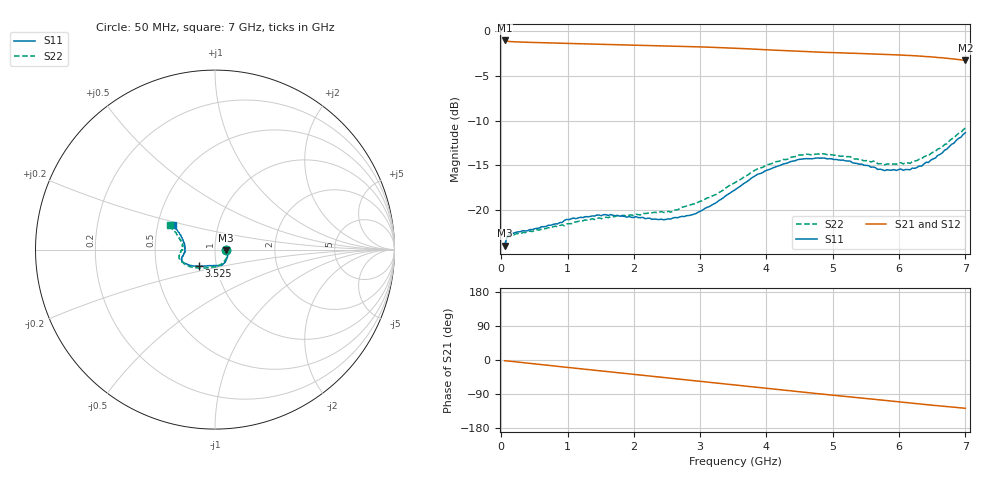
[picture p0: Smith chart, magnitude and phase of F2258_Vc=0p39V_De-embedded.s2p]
! Integrated Device Technology
! Corporate Headquarters
! 6024 Silver Creek Valley Road
! San Jose, CA 95138  USA
! Phone:  1-408-284-8200
! Toll Free:  1-800-223-1366
! Webpage:  http://www.idt.com/
! Timing and RF Division
! 515 Groton Road, Suite 102
! Westford, MA 01886-6024
! Device:  F2258
! Description: Voltage Variable RF Attenuator
! Frequency:  50.0 -  6000.00 MHz
! Package:  3x3 mm Thin QFN Plastic Package: 16 pin
! Ports:  2 RF, 2 DC
!  Pin  1  = NC
!  Pin  2  = NC
!  Pin  3  = RF2  = Port 2
!  Pin  4  = GND
!  Pin  5  = Vdd
!  Pin  6  = NC
!  Pin  7  = VCTRL
!  Pin  8  = NC
!  Pin  9  = GND
!  Pin 10  = RF1  = Port 1
!  Pin 11  = NC
!  Pin 12  = NC
!  Pin 13  = NC
!  Pin 14  = NC
!  Pin 15  = NC
!  Pin 16  = NC
! Vcntrl:  0.390 Volts
! Vdd:  +3.300 Volts
! Current:  1.093 mA
! Data:  The device was measured on a the F2258 evaluation board which has
!  individual transmission lines to the RF pins.  Data was collected
!  using a calibrated network analyzer.  The evaluation board was
!  de-embedded using a TRL calibration technique.
!  The reference plane is the edge of the package pin.
! Misc:  SN 10
!  Action Tracker AT0285
! Date Measured:  2014-12-10
! Date:  2016-01-13  MJV
! Note:
!  Integrated Device Technology supplies this data as a sample of measured
!  data at the package pin for this product.  Your particular data for this
!  product may vary.
!  Data was taken at 25 degrees C.
!  Integrated Device Technology reserves the right to change this data at anytime.
!Freq_(GHz)  S11M_(dB)  S11P_(deg)  S21M_(dB)  S21P_(deg)  S12M_(dB)  S12P_(deg)  S22M_(dB)  S22P_(deg)
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# GHz S dB R 50
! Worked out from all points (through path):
!   201 points, 50 MHz to 7 GHz, reference 50 ohm
!   highest |S21| = -1.01 dB at 50 MHz (marker M1); lowest = -3.3 dB at 7 GHz (marker M2)
!   group delay of S21, straight-line fit = 50.5 ps
!   lowest |S11| = -24.0 dB at 50 MHz (marker M3), VSWR 1.13, Z = 56.7 - j0.417 ohm
!   |S11| at or under -10 dB: start of sweep to end of sweep
!   |S22| runs from -24.1 to -10.8 dB; largest |S21 - S12| = 0.00031
!   S11 on the Smith chart (normalised r, x): 50 MHz: 1.13, -0.01; 3.525 GHz: 0.82, -0.15; 7 GHz: 0.60, +0.18
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0.05  -24.00 -3.3  -1.01 -1.9  -1.02 -2.0  -24.06 -3.0
0.08475  -23.06 -5.5  -1.09 -2.5  -1.10 -2.5  -23.14 -5.2
0.15425  -22.58 -8.6  -1.15 -3.6  -1.15 -3.6  -22.78 -9.0
0.71025  -21.71 -34.8  -1.28 -14.1  -1.28 -14.1  -21.98 -37.2
0.98825  -21.06 -48.2  -1.34 -19.4  -1.34 -19.4  -21.56 -52.8
1.2315  -20.86 -56.2  -1.39 -23.8  -1.39 -23.8  -21.22 -61.7
1.6485  -20.53 -67.6  -1.48 -31.4  -1.48 -31.4  -20.77 -74.8
2.37825  -21.09 -88.2  -1.61 -44.8  -1.61 -44.8  -20.28 -92.8
2.552  -21.03 -94.1  -1.64 -48.0  -1.64 -48.0  -20.25 -98.1
2.93425  -20.41 -110.9  -1.72 -55.1  -1.72 -55.1  -19.32 -111.6
3.247  -19.16 -123.9  -1.80 -61.0  -1.80 -61.0  -18.25 -123.9
3.525  -17.75 -134.7  -1.88 -66.2  -1.88 -66.2  -16.94 -134.5
4.0115  -15.53 -149.0  -2.06 -75.2  -2.06 -75.2  -14.93 -150.1
4.46325  -14.39 -157.7  -2.22 -83.4  -2.23 -83.4  -13.91 -161.4
4.7065  -14.25 -161.0  -2.30 -87.7  -2.30 -87.7  -13.80 -165.7
5.2625  -14.53 -167.9  -2.45 -97.4  -2.45 -97.4  -14.04 -173.8
5.6795  -15.47 -174.5  -2.53 -104.6  -2.53 -104.6  -14.83 -179.3
5.85325  -15.54 -178.7  -2.59 -107.8  -2.59 -107.8  -14.87 176.0
6.166  -15.50 173.5  -2.69 -113.4  -2.70 -113.4  -14.78 170.0
6.33975  -15.10 166.9  -2.78 -116.5  -2.78 -116.5  -14.26 165.7
6.722  -13.18 154.8  -3.01 -123.1  -3.01 -123.1  -12.59 156.6
7  -11.35 149.1  -3.26 -127.4  -3.26 -127.4  -10.82 151.6
